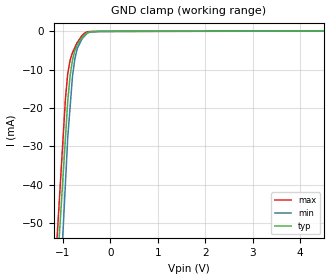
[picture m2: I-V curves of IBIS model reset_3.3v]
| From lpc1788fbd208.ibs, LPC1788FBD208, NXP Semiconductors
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[Model] reset_3.3v
Model_type Input
Vinl = 990.000mV
Vinh = 2.31000V
C_comp 1.640pF 1.560pF 1.720pF
| variable typ   min   max
[Voltage Range] 3.30000V 3.00000V 3.60000V
[POWER Clamp Reference] 3.30000V 3.00000V 3.60000V
[GND Clamp Reference] 0.00000V 0.00000V 0.00000V
[Temperature Range]   25   85   -40
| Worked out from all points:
|   GND clamp passes 1 mA (typ) near -0.54 V on its own axis
[GND Clamp]
-3.3V     -492.7mA   -615.2mA   -500.8mA
-950mV    -28.03mA   -39.91mA   -17.83mA
-900mV    -18.14mA   -27.67mA   -11.01mA
-850mV    -11.62mA   -19.71mA   -7.541mA
-800mV    -7.476mA   -11.75mA   -5.604mA
-750mV    -5.061mA   -7.22mA    -4.277mA
-700mV    -3.573mA   -4.561mA   -2.951mA
-600mV    -1.675mA   -2.009mA   -1.172mA
-500mV    -485.5uA   -671.3uA   -230uA
-400mV    -180.6uA   -127.7uA   -100.2uA
-200mV    -74.44uA   -47.52uA   -76.52uA
6.6V      153uA      31.84uA    34.45uA
[POWER Clamp]
-3.3V     0A         0A         0A
6.6V      0A         0A         0A
